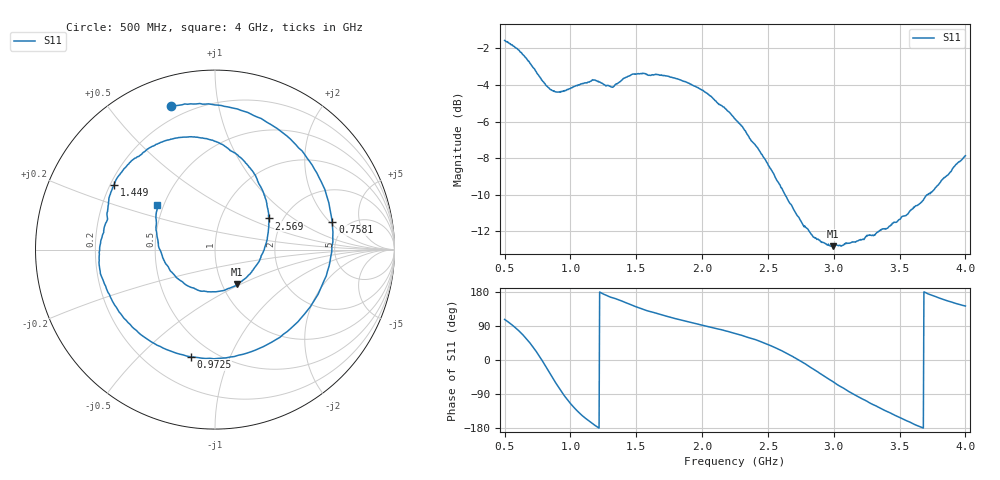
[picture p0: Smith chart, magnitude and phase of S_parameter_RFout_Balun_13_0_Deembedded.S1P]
!Agilent Technologies,E5071B,MY42403504,A.06.51
!Date: Wed Feb 26 14:57:52 2014
!Data & Calibration Information:
!Freq	S11:SOLT1(ON)
# Hz S dB R 50
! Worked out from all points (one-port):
!   801 points, 500 MHz to 4 GHz, reference 50 ohm
!   lowest |S11| = -12.8 dB at 2.994 GHz (marker M1), VSWR 1.59, Z = 59 - j23.9 ohm
!   |S11| at or under -10 dB: 2.631 GHz to 3.712 GHz (1.081 GHz wide, 34.1 % of centre)
!   S11 on the Smith chart (normalised r, x): 500 MHz: 0.14, +0.73; 758.1 MHz: 3.84, +2.13; 972.5 MHz: 0.38, -0.73; 1.449 GHz: 0.21, +0.28; 2.569 GHz: 1.69, +0.67; 4 GHz: 0.46, +0.27
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5e8  -1.56 107.0
5.74375e8  -1.90 87.5
6.35625e8  -2.32 67.6
6.925e8  -2.81 44.9
7.58125e8  -3.46 13.1
8.0625e8  -3.92 -13.3
8.5875e8  -4.29 -43.6
8.98125e8  -4.39 -65.8
9.375e8  -4.35 -86.2
9.725e8  -4.26 -102.8
1.055625e9  -4.01 -135.8
1.1475e9  -3.81 -162.6
1.248125e9  -3.95 174.4
1.375e9  -3.82 157.6
1.449375e9  -3.49 147.3
1.57625e9  -3.43 130.7
1.8125e9  -3.66 107.9
2.0225e9  -4.39 90.0
2.25e9  -5.85 69.9
2.569375e9  -9.23 30.1
2.6875e9  -10.69 9.3
2.840625e9  -12.26 -23.1
2.99375e9  -12.81 -57.0
3.125e9  -12.64 -85.3
3.34375e9  -12.00 -125.2
3.5625e9  -11.06 -161.5
3.71125e9  -10.00 175.5
4e9  -7.86 142.5
